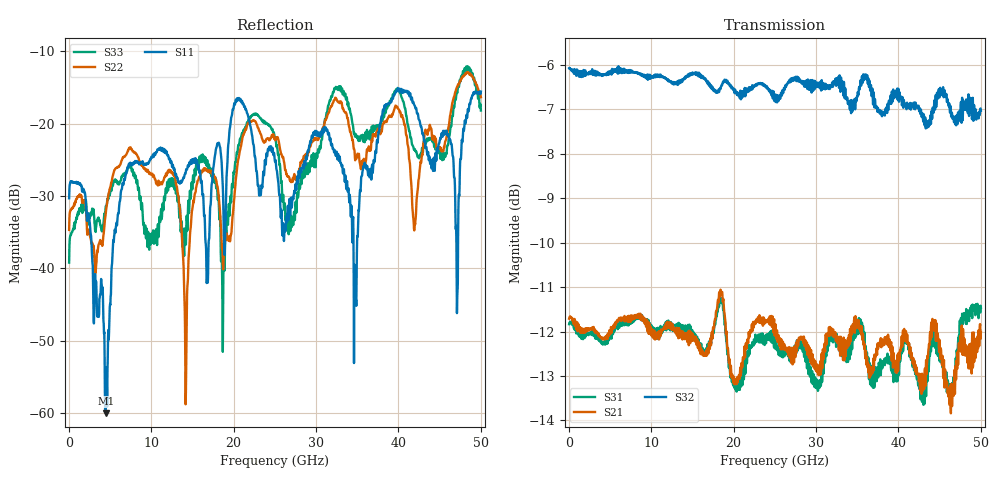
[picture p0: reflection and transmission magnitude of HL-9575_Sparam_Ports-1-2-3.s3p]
# GHZ S RI R 50.0
!; PortSelection: Port_123
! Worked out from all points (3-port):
!   1429 points, 35 MHz to 50.02 GHz, reference 50 ohm
!   strongest paths, dB at 35 MHz, 12.53 GHz, 25.02 GHz, 37.52 GHz, 50.02 GHz:
!     S32: -6.1, -6.4, -6.7, -7.0, -7.0
!     S21: -11.7, -12.0, -12.0, -12.4, -12.0
!     S31: -11.8, -11.9, -12.2, -12.8, -11.5
!   lowest |S11| = -60.1 dB at 4.48 GHz (marker M1), VSWR 1.00, Z = 50.1 - j0.0158 ohm
!   |S11| at or under -10 dB: start of sweep to end of sweep
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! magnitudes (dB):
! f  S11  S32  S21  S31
! 35 MHz  -30.3  -6.1  -11.7  -11.8
! 4.48 GHz  -60.1  -6.2  -12.1  -12.2
! 7.315 GHz  -25.5  -6.1  -11.8  -11.7
! 14.21 GHz  -26.6  -6.3  -12.2  -12.0
! 16.03 GHz  -28.1  -6.3  -12.4  -12.3
! 25.02 GHz  -25.2  -6.7  -12.0  -12.2
! 34.83 GHz  -44.7  -6.8  -11.8  -11.9
! 38.36 GHz  -17.7  -7.1  -12.1  -12.8
! 47.15 GHz  -44.0  -7.3  -12.8  -12.5
! 50.02 GHz  -15.6  -7.0  -12.0  -11.5
